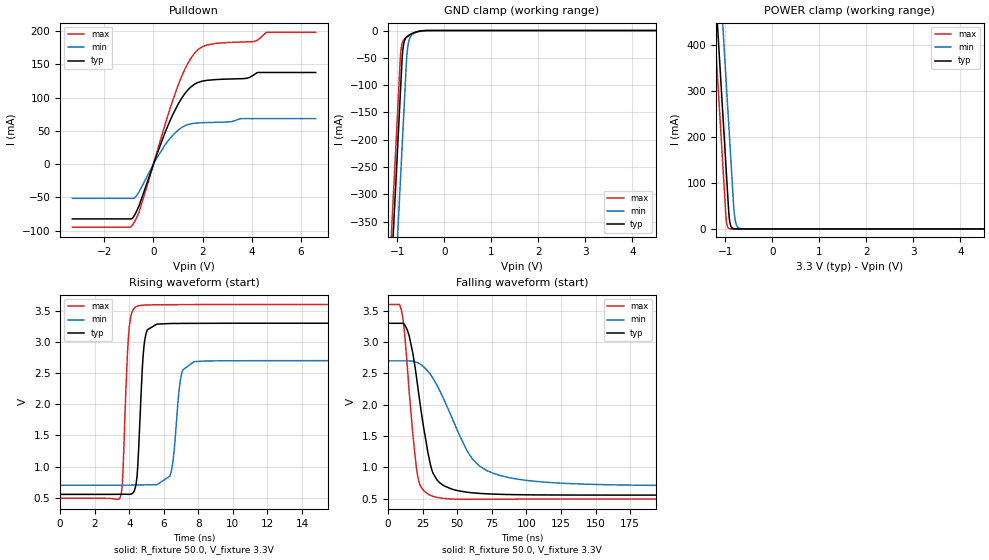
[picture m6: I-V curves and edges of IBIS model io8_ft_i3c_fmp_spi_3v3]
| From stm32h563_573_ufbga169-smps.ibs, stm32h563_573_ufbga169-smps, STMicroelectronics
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[Model]   io8_ft_i3c_fmp_spi_3v3
Model_type I/O_open_drain
Polarity   Non-Inverting
Enable   Active-Low
| CAP_THRESHOLD on pad IOFT is "UDTCAPC" :
| Rising=20.0% of vddiom   Falling=80.0% of vddiom
| C_comp min and max val. don't necessarily correlate with the min and max pvt
| but are the smallest and greatest pad capacitance found.
| var   typ   min   max
C_comp   3.95478pF  3.94672pF  4.00401pF
|C_comp_pulldown   3.95478pF  3.94672pF  4.00401pF
Vinl = 1.35V
Vinh = 1.8V
Vmeas = 1.65V   | Reference voltage for timing measurements
Cref  = 50.0pF   | Timing specification test load capacitance value
Rref  = 1.0MOhm   | Timing specification test load resistance value
Vref  = 1.815V   | Timing specification test load voltage
[Model Spec]
| TIME_THRESHOLD on pin ZII2CV11 is "CMOS" :
| Rising=40.0% of vdd   Falling=60.0% of vdd
Vinl 1.29880V 1.07480V 1.40680V
Vinh 1.77520V 1.49320V 1.89720V
| variable   typ   min   max
[Temperature Range] 25.0 125.0 -40.0
| variable   typ   min   max
[Voltage Range] 3.3V 2.7V 3.6V
| variable   typ   min   max
[POWER Clamp Reference] 3.3V 2.7V 3.6V
| variable   typ   min   max
[GND Clamp Reference] 0V 0V 0V
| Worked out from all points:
|   slope of the pulldown table from 0 to 0.495 V, typ, clamps not added: 10 ohm
|   GND clamp passes 1 mA (typ) near -0.52 V on its own axis
|   POWER clamp passes 1 mA (typ) near -0.84 V on its own axis
|   rising waveform, R_fixture 50.0, V_fixture 3.3V: 20-80 % time 285ps typ, 382ps min, 266ps max; typ from 0.556 V to 3.3 V
|   falling waveform, R_fixture 50.0, V_fixture 3.3V: 20-80 % time 11.6ns typ, 26.7ns min, 7.29ns max; typ from 3.3 V to 0.556 V
[POWER Clamp]
-3.3V     4.068A     4.259A     3.957A
-1.25V    582.8mA    774.2mA    471.5mA
-1.21V    514.8mA    706.2mA    403.5mA
-1.13V    378.8mA    570.2mA    267.5mA
-1.04V    225.8mA    417.2mA    114.5mA
-980mV    123.8mA    315.2mA    17.95mA
-920mV    26.3mA     213.2mA    906uA
-880mV    5.543mA    145.2mA    123.7uA
-810mV    363.5uA    33.6mA     3.798uA
-770mV    76.62uA    10.47mA    519.4nA
-690mV    3.409uA    1.017mA    10.46nA
6.6V      0A         0A         0A
[GND Clamp]
-3.3V     -4.13A     -4.291A    -4.063A
-1.25V    -644.7mA   -806.4mA   -578.1mA
-940mV    -117.7mA   -279.4mA   -51.06mA
-920mV    -83.75mA   -245.4mA   -31.43mA
-900mV    -50.5mA    -211.4mA   -23.14mA
-880mV    -31.27mA   -177.4mA   -19.1mA
-850mV    -18.68mA   -126.4mA   -15.73mA
-800mV    -11.46mA   -46.4mA    -12.03mA
-760mV    -8.752mA   -20.02mA   -9.606mA
-680mV    -5.122mA   -6.673mA   -5.579mA
-300mV    -5.379uA   -47.63uA   -852.7nA
6.6V      10.49nA    1.843uA    393.6pA
| variable   typ   min   max
[Pullup Reference] 3.3V 2.7V 3.6V
| variable   typ   min   max
[Pulldown Reference] 0V 0V 0V
[Pulldown]
-3.3V     -82.42mA   -51.49mA   -94.82mA
-850mV    -81.27mA   -51.49mA   -91.26mA
-580mV    -62.01mA   -41.36mA   -71.41mA
120mV     12.61mA    7.999mA    15.37mA
800mV     75.3mA     43.94mA    97.52mA
1.33V     108.3mA    58.37mA    146.5mA
1.84V     123.1mA    61.83mA    172.7mA
2.51V     126.9mA    62.69mA    181.3mA
3.78V     128.8mA    68.32mA    183.7mA
4.12V     134.9mA    68.32mA    184.6mA
4.59V     137.6mA    68.32mA    198mA
6.6V      137.6mA    68.32mA    198mA
[Ramp]
dV/dt_r 1.64663V/283.11696ps 1.19796V/378.87596ps 1.86385V/262.84369ps
dV/dt_f 1.64665V/11.53748ns 1.19674V/26.45167ns 1.86387V/7.27337ns
R_load = 50.0
| Removed startup time: 0s 0s 0s  .
| Removed end time: 34.4ns.
[Rising Waveform]
R_fixture   = 50.0
V_fixture   = 3.3V
V_fixture_min = 2.7V
V_fixture_max = 3.6V
0s        555.6mV    703.3mV    493.6mV
3.5ns     557mV      703.5mV    527.9mV
4ns       556.6mV    704.1mV    3.234V
4.5ns     1.043V     705.7mV    3.576V
4.9ns     3.033V     707.8mV    3.591V
5.6ns     3.286V     711.2mV    3.595V
6.4ns     3.295V     891.1mV    3.597V
7ns       3.297V     2.448V     3.598V
7.75ns    3.298V     2.684V     3.599V
34.4ns    3.3V       2.7V       3.6V
| Removed startup time: 0s 0s 0s  .
| Removed end time: 249.4ns.
[Falling Waveform]
R_fixture   = 50.0
V_fixture   = 3.3V
V_fixture_min = 2.7V
V_fixture_max = 3.6V
0s        3.3V       2.7V       3.6V
9.85ns    3.3V       2.7V       3.485V
15.25ns   3.1V       2.7V       2.209V
20.95ns   2.373V     2.675V     924.5mV
28.75ns   1.242V     2.537V     573.2mV
32.6ns    900.2mV    2.416V     535.9mV
40.75ns   701mV      2.066V     501.8mV
58.75ns   597.8mV    1.204V     488.3mV
76.35ns   571.6mV    901.2mV    490.2mV
249.4ns   555.6mV    705.4mV    493.6mV
